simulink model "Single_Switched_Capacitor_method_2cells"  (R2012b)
settings: Solver=ode4  StartTime=0.0  StopTime=500  FixedStep=0.000015  RelTol=1e-3
undefined symbols (not defined in the file or in its folder): InitialSOC

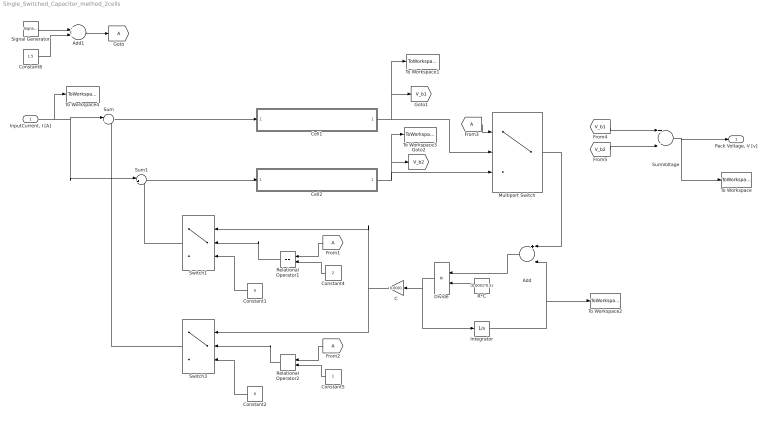
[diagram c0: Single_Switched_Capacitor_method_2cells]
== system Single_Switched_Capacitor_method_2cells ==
  "InputCurrent, I [A]" : Inport
  Add : Sum  Inputs=+-
  Add1 : Sum
  C : Gain  Gain=0.0001
  Cell1 : Subsystem
  Cell2 : Subsystem
  Constant1 : Constant  Value=0
  Constant2 : Constant  Value=0
  Constant4 : Constant  Value=2
  Constant5 : Constant
  Constant6 : Constant  Value=1.5
  Divide : Product  Inputs=*/
  From1 : From
  From2 : From
  From3 : From
  Integrator : Integrator
  Multiport Switch : MultiPortSwitch  Inputs=2
  R*C : Constant  Value=(0.0001*0.5)
  Relational Operator1 : RelationalOperator  Operator===  OutDataTypeStr=boolean
  Relational Operator2 : RelationalOperator  Operator===  OutDataTypeStr=boolean
  Signal Generator : SignalGenerator  WaveForm=square  Amplitude=0.5  Frequency=10000
  Sum : Sum  Inputs=|+-
  Sum1 : Sum  Inputs=|+-
  SumVoltage : Sum
  Switch1 : Switch  Criteria=u2 > Threshold
  Switch3 : Switch  Criteria=u2 > Threshold
  To Workspace : ToWorkspace  VariableName=PackVoltage  SampleTime=-1  SaveFormat=Structure With Time
  To Workspace1 : ToWorkspace  VariableName=CellVoltage1  SampleTime=-1  SaveFormat=Structure With Time
  To Workspace2 : ToWorkspace  VariableName=CapVoltage  SampleTime=-1  SaveFormat=Structure With Time
  To Workspace3 : ToWorkspace  VariableName=CellVoltage2  SampleTime=-1  SaveFormat=Structure With Time
  To Workspace4 : ToWorkspace  VariableName=InputCurrent  SampleTime=-1  SaveFormat=Structure With Time
  "Pack Voltage, V [v]" : Outport
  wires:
  "InputCurrent, I [A]"/1 -> To Workspace4/1, Sum1/1, Sum/1
  Cell1/1("OutputVoltage, V_b [v]") -> Multiport Switch/2, [V_b1], To Workspace1/1
  Cell2/1("OutputVoltage, V_b [v]") -> To Workspace3/1, [V_b2], Multiport Switch/3
  Switch3/1 -> Sum/2
  SumVoltage/1 -> To Workspace/1, "Pack Voltage, V [v]"/1
  Integrator/1 -> Add/2, To Workspace2/1
  Add/1 -> Divide/1
  R*C/1 -> Divide/2
  Divide/1 -> Integrator/1, C/1
  Multiport Switch/1 -> Add/1
  Sum1/1 -> Cell2/1("InputCurrent, I_b [A]")
  Sum/1 -> Cell1/1("InputCurrent, I_b [A]")
  From3/1 -> Multiport Switch/1
  Switch1/1 -> Sum1/2
  Add1/1 -> [A]
  Constant4/1 -> Relational Operator1/2
  From1/1 -> Relational Operator1/1
  Relational Operator1/1 -> Switch1/2
  Constant5/1 -> Relational Operator2/2
  From2/1 -> Relational Operator2/1
  Relational Operator2/1 -> Switch3/2
  [V_b1] -> SumVoltage/1
  [V_b2] -> SumVoltage/2
  Constant1/1 -> Switch1/3
  Constant2/1 -> Switch3/3
  C/1 -> Switch3/1, Switch1/1
  Constant6/1 -> Add1/2
  Signal Generator/1 -> Add1/1

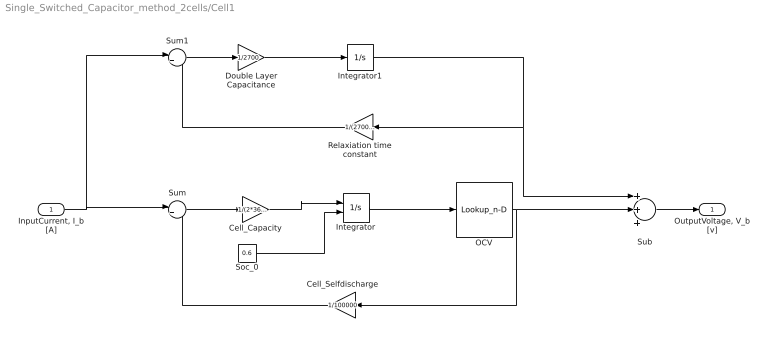
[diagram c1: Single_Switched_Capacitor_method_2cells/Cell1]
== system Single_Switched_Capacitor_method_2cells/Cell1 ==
  "InputCurrent, I_b [A]" : Inport
  Cell_Capacity : Gain  Gain=1/(2*3600)
  Cell_Selfdischarge : Gain  Gain=1/100000
  Double Layer Capacitance : Gain  Gain=1/2700
  Integrator : Integrator  InitialConditionSource=external  InitialCondition=InitialSOC
  Integrator1 : Integrator
  OCV : Lookup_n-D  NumberOfTableDimensions=1  BreakpointsForDimension1=[0 0.1 0.2 0.3 0.4 0.5 0.6 0.7 0.8 0.9 1]  Table=[2.25 3.2 3.25 3.25 3.3 3.3 3.3 3.35 3.35 3.35 3.75]  RndMeth=Simplest
  Relaxiation time constant : Gain  Gain=1/(2700*0.011)
  Soc_0 : Constant  Value=0.6
  Sub : Sum  Inputs=+++
  Sum : Sum  Inputs=|+-
  Sum1 : Sum  Inputs=|+-
  "OutputVoltage, V_b [v]" : Outport
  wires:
  Integrator/1 -> OCV/1
  OCV/1 -> Cell_Selfdischarge/1, Sub/2
  "InputCurrent, I_b [A]"/1 -> Sum1/1, Sum/1
  Cell_Capacity/1 -> Integrator/1
  Cell_Selfdischarge/1 -> Sum/2
  Integrator1/1 -> Relaxiation time constant/1, Sub/1
  Relaxiation time constant/1 -> Sum1/2
  Sub/1 -> "OutputVoltage, V_b [v]"/1
  Sum/1 -> Cell_Capacity/1
  Double Layer Capacitance/1 -> Integrator1/1
  Sum1/1 -> Double Layer Capacitance/1
  Soc_0/1 -> Integrator/2

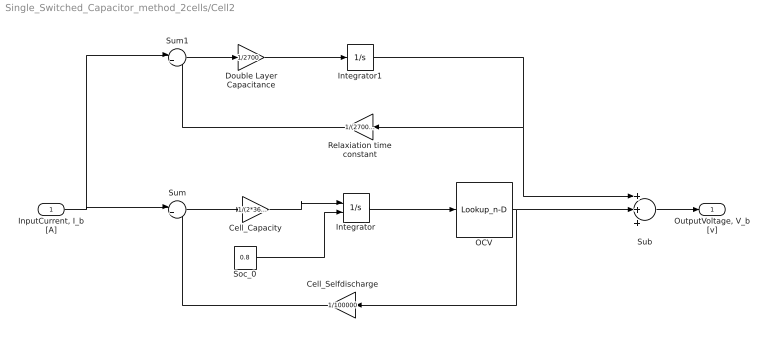
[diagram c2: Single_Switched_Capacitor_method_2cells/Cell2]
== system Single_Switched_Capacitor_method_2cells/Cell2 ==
  "InputCurrent, I_b [A]" : Inport
  Cell_Capacity : Gain  Gain=1/(2*3600)
  Cell_Selfdischarge : Gain  Gain=1/100000
  Double Layer Capacitance : Gain  Gain=1/2700
  Integrator : Integrator  InitialConditionSource=external  InitialCondition=InitialSOC
  Integrator1 : Integrator
  OCV : Lookup_n-D  NumberOfTableDimensions=1  BreakpointsForDimension1=[0 0.1 0.2 0.3 0.4 0.5 0.6 0.7 0.8 0.9 1]  Table=[2.25 3.2 3.25 3.25 3.3 3.3 3.3 3.35 3.35 3.35 3.75]  RndMeth=Simplest
  Relaxiation time constant : Gain  Gain=1/(2700*0.011)
  Soc_0 : Constant  Value=0.8
  Sub : Sum  Inputs=+++
  Sum : Sum  Inputs=|+-
  Sum1 : Sum  Inputs=|+-
  "OutputVoltage, V_b [v]" : Outport
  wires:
  Integrator/1 -> OCV/1
  OCV/1 -> Cell_Selfdischarge/1, Sub/2
  "InputCurrent, I_b [A]"/1 -> Sum1/1, Sum/1
  Cell_Capacity/1 -> Integrator/1
  Cell_Selfdischarge/1 -> Sum/2
  Integrator1/1 -> Relaxiation time constant/1, Sub/1
  Relaxiation time constant/1 -> Sum1/2
  Sub/1 -> "OutputVoltage, V_b [v]"/1
  Sum/1 -> Cell_Capacity/1
  Double Layer Capacitance/1 -> Integrator1/1
  Sum1/1 -> Double Layer Capacitance/1
  Soc_0/1 -> Integrator/2
